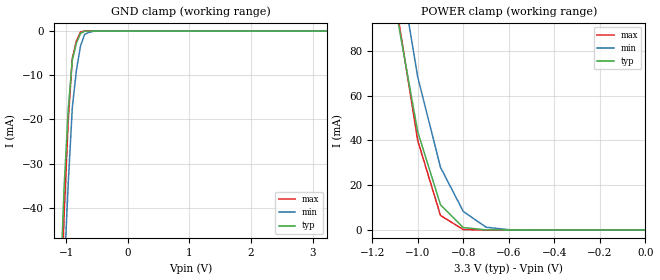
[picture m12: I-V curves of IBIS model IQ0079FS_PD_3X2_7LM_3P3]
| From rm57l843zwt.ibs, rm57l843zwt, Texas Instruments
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|   Model Cell 079FS_PD_3X2_7LM_3P3
|IQ0079FS_PD_3X2_7LM_3P3
[Model]   IQ0079FS_PD_3X2_7LM_3P3
Model_type   Input
Polarity   Non-Inverting
Vinl =  1.25
Vinh =  1.65
C_comp   1.2p   1.2p   1.2p
[Model Spec]
Vinl   1.25   1.12   1.38
Vinh   1.65   1.45   1.75
[Temperature Range]   25   155   -40
[Voltage Range]   3.3   2.97   3.63
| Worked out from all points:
|   GND clamp passes 1 mA (typ) near -0.78 V on its own axis
|   POWER clamp passes 1 mA (typ) near -0.79 V on its own axis
[POWER_clamp]
|   voltage   I(typ)   I(min)   I(max)
-3.3V     1.823A     2.351A     1.96A
-1.1V     100.7mA    129.7mA    103.9mA
-1.067V   81.76mA    109.2mA    82.61mA
-1.033V   62.81mA    88.77mA    61.28mA
-1V       43.87mA    68.31mA    39.95mA
-900mV    11.27mA    27.96mA    6.481mA
-800mV    1.099mA    8.283mA    176.7uA
-700mV    35.91uA    1.232mA    3.424uA
-600mV    1.374uA    111.2uA    455.2nA
0V        175pA      247.2pA    192.5pA
[GND_clamp]
|   voltage   I(typ)   I(min)   I(max)
-3.3V     -1.38A     -1.323A    -2.074A
-1.1V     -59.59mA   -79.11mA   -70.71mA
-1.033V   -35.48mA   -55.25mA   -41.82mA
-966.7mV  -17.81mA   -34.65mA   -20.29mA
-900mV    -6.579mA   -17.32mA   -6.122mA
-833.3mV  -2.708mA   -8.853mA   -2.234mA
-766.7mV  -527.2uA   -3.335mA   -196uA
-700mV    -37.17uA   -765.8uA   -8.209uA
-566.7mV  -1.613uA   -62.15uA   -984.8nA
3.233V    168.9pA    53.88nA    156.8pA
